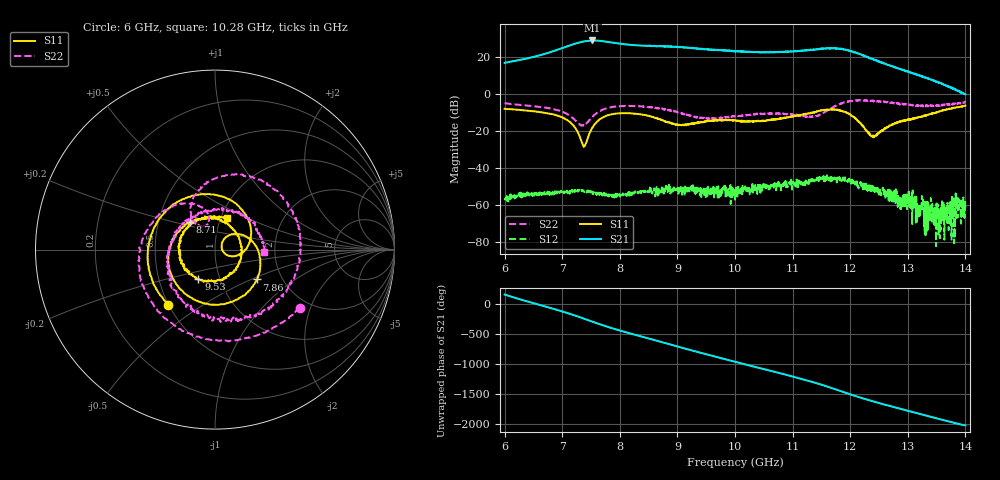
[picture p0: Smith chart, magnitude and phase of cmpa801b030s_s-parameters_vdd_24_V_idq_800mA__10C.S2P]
!Keysight Technologies,E5071C,MY46110325,B.14.03
!Date: Fri Aug 07 13:51:34 2020
!Data & Calibration Information:
!Freq	S11:SOLT2(ON)	S21:SOLT2(ON)	S12:SOLT2(ON)	S22:SOLT2(ON)
!PortZ  Port1:50+j0  Port2:50+j0
!Above PortZ is port z conversion or system Z0 setting when saving the data.
!When reading, reference impedance value at option line is always used.
# Hz S dB R 50
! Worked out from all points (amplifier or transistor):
!   1601 points, 6 GHz to 14 GHz, reference 50 ohm
!   highest |S21| = 29.1 dB at 7.525 GHz (marker M1)
!   |S21| within 3 dB of that: 7.103 GHz to 8.541 GHz (1.438 GHz wide, 18.4 % of centre)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
!   unconditionally stable (mu >= 1): start of sweep to end of sweep
!   at 7.33 GHz: K = 7.36, MAG = 28.4 dB, |S12| = -51.8 dB
!   at 10 GHz: K = 22.09, MAG = 23.8 dB, |S12| = -57.2 dB
!   at 14 GHz: K = 350.14, MAG = 3.2 dB, |S12| = -63.4 dB
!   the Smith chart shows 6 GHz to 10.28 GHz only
!   S11 on the Smith chart (normalised r, x): 6 GHz: 0.50, -0.36; 7.86 GHz: 1.49, -0.54; 8.71 GHz: 0.72, +0.23; 9.53 GHz: 0.79, -0.27; 10.28 GHz: 1.07, +0.39
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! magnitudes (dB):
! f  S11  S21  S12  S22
! 6 GHz  -7.9  17.0  -56.6  -4.8
! 6.995 GHz  -12.4  24.9  -53.5  -9.5
! 7.2 GHz  -17.2  27.1  -52.9  -13.2
! 7.335 GHz  -25.7  28.4  -52.1  -16.9
! 7.4 GHz  -27.4  28.7  -52.9  -16.4
! 7.525 GHz  -18.0  29.1  -54.0  -12.4
! 7.86 GHz  -10.8  28.0  -55.4  -7.0
! 8.67 GHz  -13.4  26.0  -52.1  -7.6
! 8.71 GHz  -13.6  26.1  -52.8  -7.8
! 9.53 GHz  -14.4  24.2  -50.1  -13.6
! 10 GHz  -14.2  23.3  -57.2  -11.8
! 10.28 GHz  -14.6  23.0  -52.8  -11.3
! 11.34 GHz  -10.1  24.1  -45.8  -12.2
! 11.9 GHz  -9.5  24.2  -47.0  -4.4
! 12.39 GHz  -22.5  19.1  -49.6  -3.3
! 12.67 GHz  -17.4  15.8  -57.6  -4.2
! 12.97 GHz  -14.2  12.5  -53.1  -5.7
! 13.53 GHz  -9.6  6.3  -75.9  -5.9
! 13.62 GHz  -8.7  5.3  -58.2  -5.8
! 13.78 GHz  -7.5  3.5  -66.6  -5.7
! 13.87 GHz  -7.0  1.7  -66.8  -4.7
! 14 GHz  -6.1  -0.1  -63.4  -4.2
